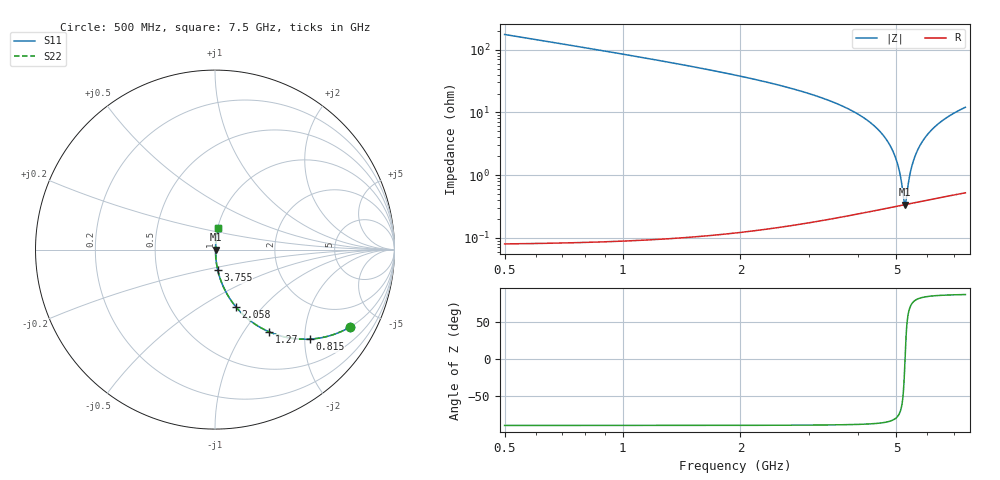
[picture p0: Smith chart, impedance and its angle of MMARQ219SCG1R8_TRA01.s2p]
! MMARQ219SCG1R8_TRA01  S-PARAMETER MODEL  ( General Type )
! Model Generated by TAIYO YUDEN Corporation (http://www.ty-top.com)
! Version 1.0
! TAIYO YUDEN Control No. 180601
! Copyright(c) 2018 TAIYO YUDEN CO.,LTD. All Rights Reserved.
! Product Description (link to TY-COMPAS)
! https://ds.yuden.co.jp/TYCOMPAS/or/detail?pn=MMARQ219SCG1R8BTRA01&u=M
! Products Name : Multilayer Ceramic Capacitors
! Characteristics :
!  Capacitance : 1.8 pF , Rated Voltage : 250V , TCC : CG / C0G
!  Case Size : 2.0 x 1.25 / 0.079 x 0.049 [mm/inch] , Thickness : 0.85 / 0.033 [mm/inch]
!  (Conditions: Temperature = 25 degC , DC Bias Current/Voltage = 0A / 0V)
! External Node Assignments :
!  1  o---| |---o  2
! GND o---------o GND
! Frequency Range : 500MHz  -  7500MHz  [ 401 STEP ]
# MHz S RI R 50
! Freq[MHz].  S11 Real  S11 Imag  S21 Real  S21 Imag  S12 Real  S12 Imag  S22 Real  S22 Imag
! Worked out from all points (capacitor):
!   401 points, 500 MHz to 7.5 GHz, reference 50 ohm
!   read as one part in series: C = 1.8 pF near 535 MHz
!   lowest |Z| = 336 mohm at 5.26 GHz (marker M1)
!   series resonance near 5.26 GHz, so ESL is about 510 pH
!   S11 on the Smith chart (normalised r, x): 500 MHz: 1.00, -3.51; 815 MHz: 1.00, -2.12; 1.27 GHz: 1.00, -1.31; 2.058 GHz: 1.00, -0.73; 3.755 GHz: 1.00, -0.23; 7.5 GHz: 1.01, +0.24
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500  0.7543 -0.4303  0.2457 0.4303  0.2457 0.4303  0.7543 -0.4303
815  0.5286 -0.4988  0.4714 0.4988  0.4714 0.4988  0.5286 -0.4988
1270  0.3008 -0.4579  0.6992 0.4579  0.6992 0.4579  0.3008 -0.4579
1672.5  0.1846 -0.3869  0.8154 0.3869  0.8154 0.3869  0.1846 -0.3869
2057.5  0.1176 -0.3205  0.8824 0.3205  0.8824 0.3205  0.1176 -0.3205
2845  0.0474 -0.2087  0.9526 0.2087  0.9526 0.2087  0.0474 -0.2087
3755  0.0152 -0.1131  0.9848 0.1131  0.9848 0.1131  0.0152 -0.1131
4000  0.0109 -0.0917  0.9891 0.0917  0.9891 0.0917  0.0109 -0.0917
4472.5  0.00568 -0.0541  0.9943 0.0541  0.9943 0.0541  0.00568 -0.0541
4805  0.0039 -0.0301  0.9961 0.0301  0.9961 0.0301  0.0039 -0.0301
5032.5  0.00339 -0.0147  0.9966 0.0147  0.9966 0.0147  0.00339 -0.0147
5102.5  0.00333 -0.0101  0.9967 0.0101  0.9967 0.0101  0.00333 -0.0101
5172.5  0.00331 -0.00558  0.9967 0.00558  0.9967 0.00558  0.00331 -0.00558
5225  0.00333 -0.00223  0.9967 0.00223  0.9967 0.00223  0.00333 -0.00223
5260  0.00335 -9.61e-06  0.9966 9.61e-06  0.9966 9.61e-06  0.00335 -9.61e-06
5295  0.00339 0.00219  0.9966 -0.00219  0.9966 -0.00219  0.00339 0.00219
5382.5  0.00351 0.00763  0.9965 -0.00763  0.9965 -0.00763  0.00351 0.00763
5452.5  0.00365 0.0119  0.9964 -0.0119  0.9964 -0.0119  0.00365 0.0119
5627.5  0.00415 0.0224  0.9958 -0.0224  0.9958 -0.0224  0.00415 0.0224
5925  0.00546 0.0395  0.9945 -0.0395  0.9945 -0.0395  0.00546 0.0395
6345  0.00813 0.0621  0.9919 -0.0621  0.9919 -0.0621  0.00813 0.0621
7500  0.0193 0.1176  0.9807 -0.1176  0.9807 -0.1176  0.0193 0.1176
